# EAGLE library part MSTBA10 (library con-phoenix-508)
PHOENIX
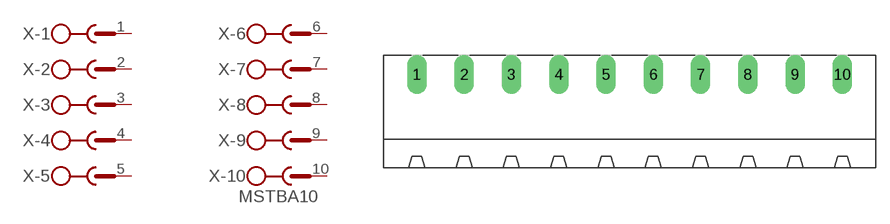
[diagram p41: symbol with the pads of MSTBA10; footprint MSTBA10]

Designator prefix X; gates -1=SK -2=SK -3=SK -4=SK -5=SK -6=SK -7=SK -8=SK -9=SK -10=SKV

## MSTBA10 (MF: FARNELL; MPN: 1757323; OC_FARNELL: 3705249; OC_NEWARK: 71C4168)  [MSTBA10]
1  -1:1  pas
2  -2:1  pas
3  -3:1  pas
4  -4:1  pas
5  -5:1  pas
6  -6:1  pas
7  -7:1  pas
8  -8:1  pas
9  -9:1  pas
10  -10:1  pas

## Footprint MSTBA10 (pad centres in mm)
PHOENIX
drill 1.397 long: 1 -22.86,5.08; 2 -17.78,5.08; 3 -12.7,5.08; 4 -7.62,5.08; 5 -2.54,5.08; 6 2.54,5.08; 7 7.62,5.08; 8 12.7,5.08; 9 17.78,5.08; 10 22.86,5.08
